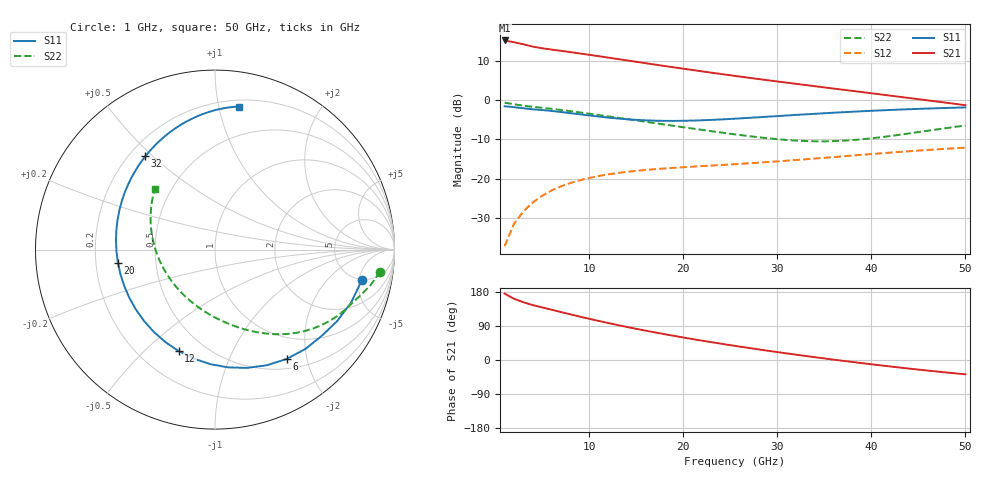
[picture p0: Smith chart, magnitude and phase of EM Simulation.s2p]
!freq-unit  param-type  data-format  keyword  impedance-ohms
# GHZ  S  MA  R  50
!Freq  MagS11  AngS11  MagS21  AngS21  MagS12  AngS12  MagS22  AngS22
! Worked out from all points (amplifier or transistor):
!   50 points, 1 GHz to 50 GHz, reference 50 ohm
!   highest |S21| = 15.2 dB at 1 GHz (marker M1)
!   |S21| within 3 dB of that: start of sweep to 8.067 GHz
!   unconditionally stable (mu >= 1): nowhere
!   at 9 GHz: K = 0.43, MSG = 16.2 dB, |S12| = -20.4 dB
!   at 26 GHz: K = 0.87, MSG = 11.1 dB, |S12| = -16.2 dB
!   at 50 GHz: K = 0.79, MSG = 5.4 dB, |S12| = -12.1 dB
!   S11 on the Smith chart (normalised r, x): 1 GHz: 4.87, -5.49; 6 GHz: 0.64, -1.66; 12 GHz: 0.36, -0.64; 20 GHz: 0.30, -0.06; 32 GHz: 0.26, +0.47; 50 GHz: 0.25, +1.15
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1  0.8359 -11.7  5.775 175.3  0.01375 88.2  0.9289 -7.7
2  0.8139 -21.2  5.479 161.6  0.0265 79.9  0.8876 -13.0
3  0.7883 -30.4  5.16 152.3  0.03823 74.7  0.8506 -17.3
4  0.7645 -38.9  4.817 144.8  0.0496 70.6  0.8225 -21.0
6  0.7285 -56.8  4.417 132.7  0.07055 61.9  0.7752 -28.6
7  0.7061 -65.8  4.257 126.5  0.07962 58.0  0.7498 -32.2
8  0.6831 -74.8  4.099 120.4  0.08784 54.3  0.7241 -35.8
10  0.6385 -92.4  3.789 108.7  0.1019 47.5  0.6726 -42.6
12  0.6003 -109.8  3.493 97.7  0.113 41.7  0.6224 -48.9
13  0.5846 -118.2  3.352 92.4  0.1177 39.1  0.5982 -52.0
15  0.5609 -134.8  3.086 82.3  0.1255 34.5  0.5522 -58.1
18  0.5448 -158.1  2.729 68.2  0.1346 28.9  0.4895 -67.1
20  0.5458 -172.3  2.519 59.4  0.1397 25.9  0.452 -73.4
23  0.5604 168.7  2.241 47.0  0.1467 22.3  0.4021 -83.7
26  0.5854 152.4  2.002 35.4  0.1541 19.4  0.36 -95.7
29  0.616 138.6  1.795 24.4  0.1627 16.9  0.3268 -109.9
32  0.6487 126.8  1.615 14.0  0.1727 14.4  0.3053 -126.5
34  0.6705 119.8  1.506 7.4  0.1801 12.6  0.2991 -138.8
38  0.7124 107.7  1.312 -5.3  0.1967 8.4  0.3096 -164.4
42  0.7501 97.4  1.143 -17.1  0.2143 3.4  0.3488 171.8
46  0.7822 88.5  0.9942 -27.9  0.2318 -2.3  0.4078 151.6
50  0.8081 80.6  0.8637 -37.7  0.2481 -8.5  0.4753 134.9
